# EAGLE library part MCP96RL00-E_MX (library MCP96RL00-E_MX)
Board Mount Temperature Sensors +/- 8.0C Thermocouple to I2C converter in 5mmx5mm QFN. This device supports K, J, T, N, S, E, B, and R type thermocouples. Source: Datasheet
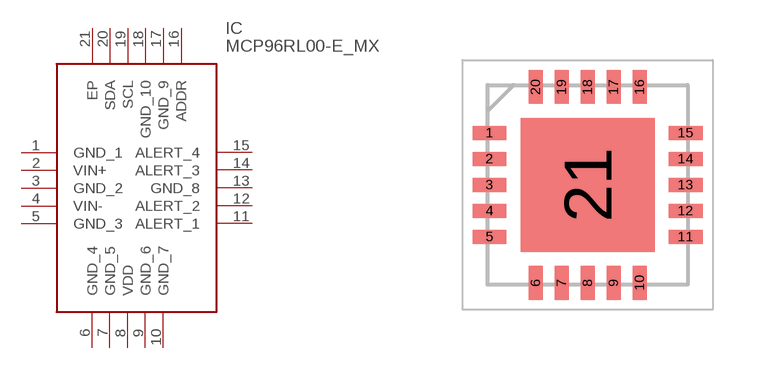
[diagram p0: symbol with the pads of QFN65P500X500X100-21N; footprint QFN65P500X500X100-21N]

Designator prefix IC

## MCP96RL00-E_MX (Description: Board Mount Temperature Sensors +/- 8.0C Thermocouple to I2C converter in 5mmx5mm QFN. This device supports K, J, T, N, S, E, B, and R type thermocouples.; Height: 1mm; Manufacturer_Name: Microchip; Manufacturer_Part_Number: MCP96RL00-E/MX; Mouser_Part_Number: 579-MCP96RL00-E/MX; Mouser_Price-Stock: https://www.mouser.co.uk/ProductDetail/Microchip-Technology/MCP96RL00-E-MX?qs=u16ybLDytRaPVbMV4dyqRg%3D%3D)  [QFN65P500X500X100-21N]
1  GND_1
2  VIN+
3  GND_2
4  VIN-
5  GND_3
6  GND_4
7  GND_5
8  VDD
9  GND_6
10  GND_7
11  ALERT_1
12  ALERT_2
13  GND_8
14  ALERT_3
15  ALERT_4
16  ADDR
17  GND_9
18  GND_10
19  SCL
20  SDA
21  EP

## Footprint QFN65P500X500X100-21N (pad centres in mm)
MCP96RL00-E/MX
smd 0.85 x 0.35: 1 -2.45,1.3; 2 -2.45,0.65; 3 -2.45,0; 4 -2.45,-0.65; 5 -2.45,-1.3; 11 2.45,-1.3; 12 2.45,-0.65; 13 2.45,0; 14 2.45,0.65; 15 2.45,1.3
smd 0.35 x 0.85: 6 -1.3,-2.45; 7 -0.65,-2.45; 8 0,-2.45; 9 0.65,-2.45; 10 1.3,-2.45; 16 1.3,2.45; 17 0.65,2.45; 18 0,2.45; 19 -0.65,2.45; 20 -1.3,2.45
smd 3.35 x 3.35: 21 0,0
